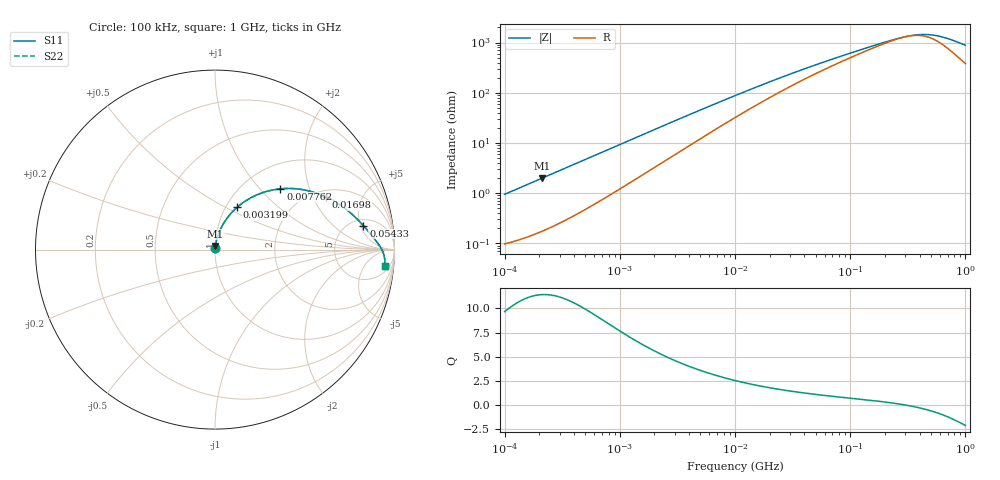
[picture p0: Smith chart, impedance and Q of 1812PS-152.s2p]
# MHz S MA R 50
!Freq  MagS11  AngS11  MagS21  AngS21  MagS12  AngS12  MagS22  AngS22
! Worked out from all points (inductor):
!   801 points, 100 kHz to 1 GHz, reference 50 ohm
!   read as one part in series: L = 1.5 uH near 104.7 kHz
!   highest Q = 11.4 at 211.3 kHz (marker M1), where L = 1.49 uH
!   self-resonance near 307.1 MHz
!   S11 on the Smith chart (normalised r, x): 100 kHz: 1.00, +0.02; 3.199 MHz: 1.13, +0.57; 7.762 MHz: 1.45, +1.30; 16.98 MHz: 2.30, +2.54; 54.33 MHz: 6.25, +5.59; 1 GHz: 9, -16
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0.1  0.009442 83.6  0.999 -0.5  0.999 -0.5  0.009442 83.6
0.2113489  0.01987 83.9  0.9981 -1.1  0.9981 -1.1  0.01987 83.9
0.4677351  0.04367 81.9  0.9948 -2.5  0.9948 -2.5  0.04367 81.9
1.047129  0.09609 77.0  0.9828 -5.5  0.9828 -5.5  0.09609 77.0
2.162719  0.1897 68.8  0.9479 -10.8  0.9479 -10.8  0.1897 68.8
3.198895  0.2665 62.3  0.9075 -15.1  0.9075 -15.1  0.2665 62.3
4.841724  0.368 53.9  0.8378 -20.8  0.8378 -20.8  0.368 53.9
7.762471  0.4971 42.9  0.7204 -28.0  0.7204 -28.0  0.4971 42.9
10  0.5646 36.9  0.6446 -31.7  0.6446 -31.7  0.5646 36.9
16.98244  0.6849 25.3  0.4807 -37.6  0.4807 -37.6  0.6849 25.3
27.54229  0.7644 17.0  0.3503 -39.8  0.3503 -39.8  0.7644 17.0
46.77351  0.8244 10.6  0.2425 -38.6  0.2425 -38.6  0.8244 10.6
54.32503  0.8377 9.2  0.2184 -37.6  0.2184 -37.6  0.8377 9.2
100  0.8806 4.8  0.1431 -31.1  0.1431 -31.1  0.8806 4.8
216.2719  0.9174 1.3  0.08547 -14.2  0.08547 -14.2  0.9174 1.3
278.6121  0.9264 0.4  0.0738 -4.5  0.0738 -4.5  0.9264 0.4
338.8442  0.9326 -0.4  0.06771 5.0  0.06771 5.0  0.9326 -0.4
402.717  0.9373 -1.0  0.06502 14.9  0.06502 14.9  0.9373 -1.0
467.7351  0.9409 -1.6  0.06514 24.1  0.06514 24.1  0.9409 -1.6
543.2503  0.944 -2.3  0.06785 33.2  0.06785 33.2  0.944 -2.3
638.2635  0.9466 -3.0  0.07383 42.2  0.07383 42.2  0.9466 -3.0
1000  0.9492 -5.6  0.1072 59.0  0.1072 59.0  0.9492 -5.6
